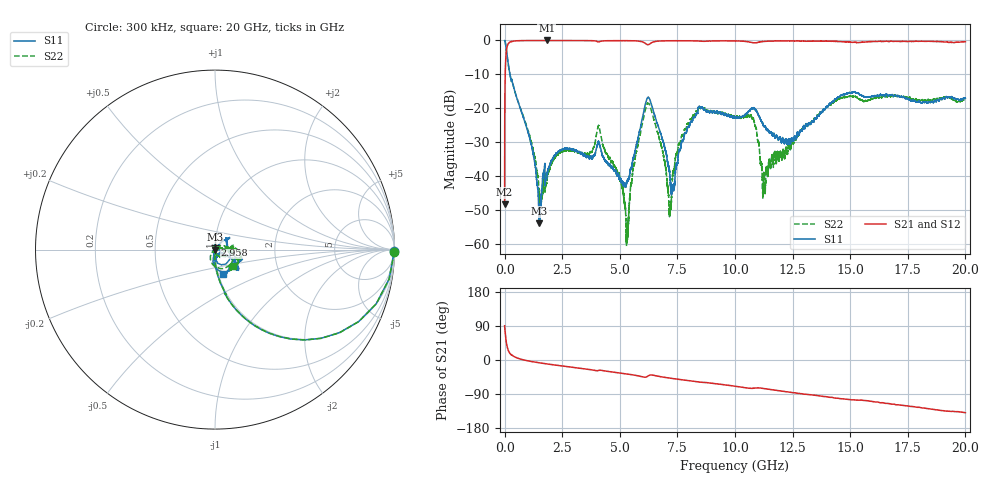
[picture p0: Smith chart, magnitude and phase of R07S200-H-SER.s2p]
!{R07S200}
!Johanson Technology Inc.
!www.johansontechnology.com
!Test Board Conditions:
!Substrate Type  RO4350B
!Substrate Thickness  10 mil
!Substrate Dk  3.66
!TL Type: GCPW
!TL Trace Width  21 mil
!TL Gap  20 mil
!Electrode orientation  Horizontal
!DUT TOPOLOGY	SERIES
!Mounting Pad LxW  16x21 mil
! Created Sat Feb  6 11:50:01 2021
# hz S ma R 50
! 2 Port Network Data from SP1.SP block
! freq  magS11  angS11  magS21  angS21  magS12  angS12  magS22  angS22
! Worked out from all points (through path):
!   20001 points, 300 kHz to 20 GHz, reference 50 ohm
!   highest |S21| = -0.01 dB at 1.833 GHz (marker M1); lowest = -48.4 dB at 300 kHz (marker M2)
!   group delay of S21, straight-line fit = 20.2 ps
!   lowest |S11| = -54.1 dB at 1.506 GHz (marker M3), VSWR 1.00, Z = 49.8 - j0.00565 ohm
!   |S11| at or under -10 dB: 233 MHz to end of sweep
!   |S22| runs from -60.8 to 0.0 dB; largest |S21 - S12| = 0.012
!   S11 on the Smith chart (normalised r, x): 300 kHz: open; 2.958 GHz: 1.00, +0.05; 20 GHz: 1.05, -0.29
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300000  0.9978 -0.6  0.003809 90.3  0.003744 89.1  1 -0.7
1.023e8  0.6096 -52.9  0.7887 37.4  0.7902 37.2  0.6113 -52.9
1.633e8  0.4325 -65.5  0.8987 24.9  0.8989 25.0  0.4323 -65.4
1.1513e9  0.02976 -96.2  0.9971 -3.8  0.9971 -3.9  0.03233 -90.4
1.5063e9  0.001978 -178.4  0.9976 -7.3  0.9976 -7.4  0.005202 -55.7
1.8333e9  0.00975 89.7  0.9989 -10.3  0.998 -10.3  0.008317 57.8
2.9583e9  0.02458 86.6  0.9956 -19.3  0.9957 -19.3  0.02402 43.1
3.3343e9  0.02137 91.7  0.9953 -22.2  0.9959 -22.2  0.02202 28.5
4.1103e9  0.02997 -55.1  0.9586 -27.1  0.9579 -27.0  0.05207 -43.9
5.0223e9  0.008911 -116.4  0.9936 -34.4  0.9925 -34.4  0.008256 -90.1
5.3113e9  0.00821 -54.5  0.9925 -36.9  0.9918 -36.9  0.001225 -13.2
6.1463e9  0.1277 -26.4  0.8865 -45.0  0.8865 -45.0  0.1057 -20.2
6.6673e9  0.0543 -100.8  0.9773 -42.9  0.9783 -43.0  0.04137 -126.5
7.1683e9  0.01042 -74.9  0.9897 -47.8  0.9886 -47.8  0.003348 -52.5
7.6093e9  0.02361 53.1  0.9901 -51.5  0.99 -51.5  0.02958 12.8
8.3733e9  0.08375 43.9  0.9822 -57.5  0.9818 -57.5  0.08923 9.3
1.00003e10  0.07373 21.8  0.9826 -69.2  0.9834 -69.2  0.07218 8.1
1.07633e10  0.09913 -42.8  0.9259 -74.8  0.9264 -74.8  0.07063 -26.8
1.12613e10  0.05409 -86.3  0.9681 -75.5  0.9696 -75.5  0.01047 170.9
1.33343e10  0.06228 -30.4  0.9744 -92.0  0.9757 -92.1  0.06346 0.5
1.66673e10  0.153 -19.3  0.9623 -114.9  0.9689 -115.2  0.1519 -36.0
2e10  0.1405 -72.3  0.9602 -139.1  0.9539 -139.0  0.1368 -42.8
